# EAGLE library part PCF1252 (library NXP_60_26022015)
Threshold detector and reset generator The PCF1252-Xs are low-power CMOS voltage threshold detectors designed especially for supervision of microcontroller/microprocessor systems for detection of power-on/off conditions and generation of a system reset pulse. The PCF1252-X also provides a POWF (power fail) output which is activated at a precise factory-programmed trip point. A system RESET output has a built-in delay with duration determined by an external capacitor (CCT). A second comparator (comparator 2) has been included to enable the possibility of a second monitoring point in the system. AAL Eindhoven MK
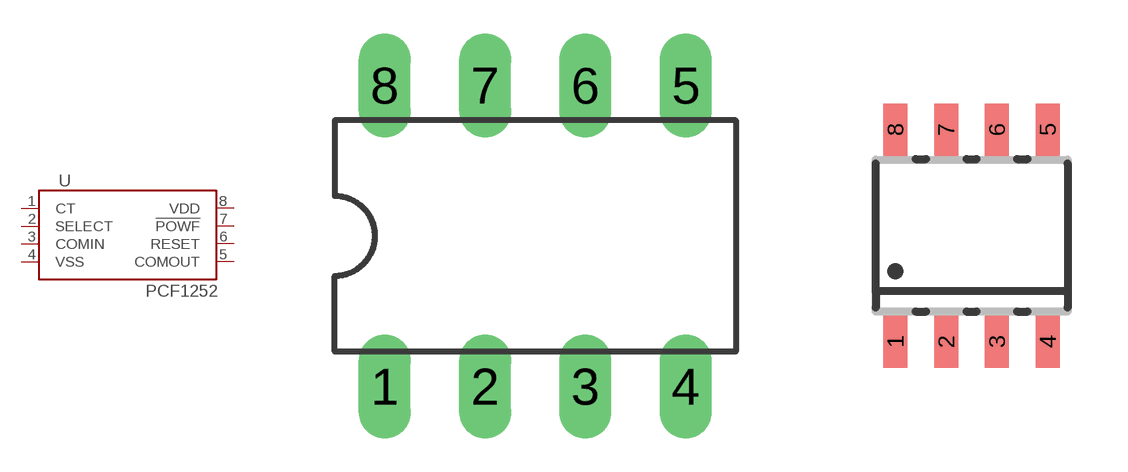
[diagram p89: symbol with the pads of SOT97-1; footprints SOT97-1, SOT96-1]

Designator prefix U

## PCF1252-0P, PCF1252-1P, PCF1252-2P, PCF1252-3P, PCF1252-4P, PCF1252-5P, PCF1252-6P, PCF1252-7P, PCF1252-8P, PCF1252-9P  [SOT97-1]
1  CT  pas
2  SELECT  in
3  COMIN  pas
4  VSS  pwr
5  COMOUT  out
6  RESET  out
7  !POWF!  out
8  VDD  pwr

## PCF1252-0T, PCF1252-1T, PCF1252-2T, PCF1252-3T, PCF1252-4T, PCF1252-5T, PCF1252-6T, PCF1252-7T, PCF1252-8T, PCF1252-9T  [SOT96-1]
Pads as for SOT97-1

## Footprint SOT97-1 (pad centres in mm)
Dual In Line Package
drill 0.813 long: 1 -3.81,-3.81; 2 -1.27,-3.81; 3 1.27,-3.81; 4 3.81,-3.81; 5 3.81,3.81; 6 1.27,3.81; 7 -1.27,3.81; 8 -3.81,3.81

## Footprint SOT96-1 (pad centres in mm)
SOT96-1 SO8: plastic small outline package; 8 leads; body width 3.9 mm JEDEC: MS-012 IEC: 076E03
smd 0.6 x 1.3: 1 -1.905,-2.65; 2 -0.635,-2.65; 3 0.635,-2.65; 4 1.905,-2.65; 5 1.905,2.65; 6 0.635,2.65; 7 -0.635,2.65; 8 -1.905,2.65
